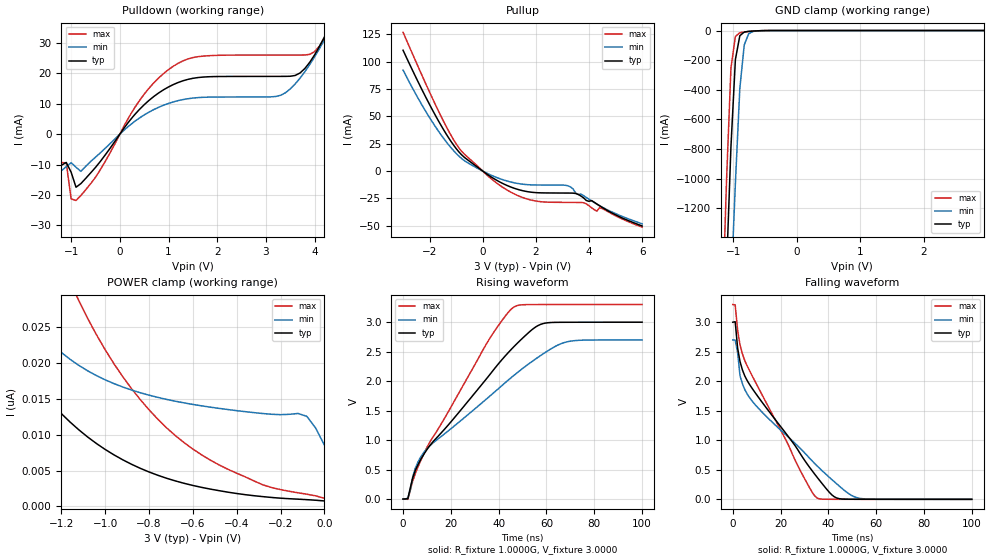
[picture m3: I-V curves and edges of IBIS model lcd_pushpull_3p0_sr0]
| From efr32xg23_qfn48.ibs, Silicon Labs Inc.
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|   Model lcd_pushpull_3p0_sr0
[Model]  lcd_pushpull_3p0_sr0
Model_type 3-state
Polarity   Non-Inverting
Enable   Active-High
C_comp   1.6300pF   1.4000pF   2.7000pF
[Temperature Range]   25.0000   0.1250k   -40.0000
[Pullup Reference]   3.0000V   2.7000V   3.3000V
[Pulldown Reference]   0.0V   0.0V   0.0V
[POWER Clamp Reference]   3.0000V   2.7000V   3.3000V
[GND Clamp Reference]   0.0V   0.0V   0.0V
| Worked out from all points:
|   slope of the pulldown table from 0 to 0.45 V, typ, clamps not added: 50.8 ohm
|   slope of the pullup table from 0 to 0.45 V, typ, clamps not added: 61.2 ohm
|   GND clamp passes 1 mA (typ) near -0.56 V on its own axis
|   rising waveform, R_fixture 1.0000G, V_fixture 3.0000: 20-80 % time 35.7ns typ, 43ns min, 27.5ns max; typ from 0 V to 3 V
|   falling waveform, R_fixture 1.0000G, V_fixture 3.0000: 20-80 % time 28.4ns typ, 33.1ns min, 23.2ns max; typ from 3 V to 0 V
[Pulldown]
|Voltage   I(typ)   I(min)   I(max)
-3V       -29.4mA    -32.34mA   -24.51mA
-1.2V     -10.22mA   -12.02mA   -9.329mA
-1.1V     -9.298mA   -10.66mA   -9.429mA
-1V       -12.5mA    -9.381mA   -21.28mA
-900mV    -17.44mA   -10.87mA   -21.78mA
-800mV    -16.24mA   -12.22mA   -20.16mA
500mV     9.663mA    6.314mA    13.13mA
1.3V      17.55mA    11.37mA    24.1mA
3.3V      18.98mA    12.75mA    25.98mA
3.9V      23.59mA    22.85mA    26.21mA
4.4V      38.7mA     37.11mA    38.07mA
6V        113.8mA    103.8mA    120mA
[Pullup]
|Voltage   I(typ)   I(min)   I(max)
-3V       110.5mA    92.37mA    126.9mA
-2V       60.77mA    48.83mA    72.09mA
-1.1V     23.81mA    18.74mA    28.76mA
-700mV    12.76mA    9.696mA    15.64mA
400mV     -6.625mA   -4.651mA   -8.607mA
1.7V      -18.89mA   -12.46mA   -25.74mA
3.2V      -20.11mA   -13.42mA   -28.65mA
3.5V      -20.5mA    -20.09mA   -28.69mA
3.8V      -24.56mA   -22.6mA    -28.98mA
4.3V      -30.18mA   -30.25mA   -36.64mA
4.5V      -33.28mA   -32.98mA   -34.28mA
6V        -50.2mA    -48.25mA   -51.3mA
[GND_clamp]
|Voltage   I(typ)   I(min)   I(max)
-3V       -24.27A    -21.95A    -26.57A
-1.18V    -2.447A    -3.183A    -1.952A
-1.11V    -1.614A    -2.464A    -1.015A
-1.04V    -784mA     -1.746A    -252.8mA
-970mV    -196.2mA   -1.031A    -40.03mA
-900mV    -35mA      -390.7mA   -14.95mA
-830mV    -10.34mA   -96.94mA   -9.948mA
-760mV    -5.711mA   -21.43mA   -6.561mA
-690mV    -3.47mA    -6.05mA    -3.879mA
-340mV    -10.36uA   -45.49uA   -3.3uA
2.95V     657.9pA    12.89nA    538.5pA
[POWER_clamp]
|Voltage   I(typ)   I(min)   I(max)
-3V       338.2nA    9.289uA    586.7nA
-1.56V    29.18nA    39.44nA    70.52nA
-1.4V     20.57nA    28.74nA    51.74nA
-1.28V    15.63nA    23.83nA    40.5nA
-1.12V    10.68nA    19.68nA    28.7nA
-1V       7.945nA    17.67nA    21.86nA
-880mV    5.879nA    16.25nA    16.45nA
-640mV    3.219nA    14.45nA    8.897nA
-280mV    1.357nA    12.96nA    2.997nA
-120mV    1.003nA    12.97nA    1.894nA
-80mV     936.4pA    12.58nA    1.698nA
0V        757.3pA    8.576nA    1.134nA
[Ramp]
| variable   typ   min   max
dV/dt_r  1.7810/38.6720n   1.5858/48.4026n   1.9678/29.1326n
dV/dt_f  1.7893/31.8128n   1.6007/39.1915n   1.9729/24.9987n
R_load = 10.0000k
[Rising Waveform]
R_fixture= 1.0000G
V_fixture= 3.0000
V_fixture_min= 2.7000
V_fixture_max= 3.3000
|time   V(typ)   V(min)   V(max)
0s        214.6uV    425.1uV    123.1uV
2.02ns    8.808mV    17.95mV    -4.717mV
5.051ns   477.2mV    514mV      424.4mV
10.1ns    845.4mV    859.4mV    883.8mV
35.35ns   2.063V     1.713V     2.663V
45.45ns   2.546V     2.067V     3.228V
48.48ns   2.67V      2.166V     3.288V
56.57ns   2.945V     2.407V     3.299V
67.68ns   2.998V     2.657V     3.299V
100ns     2.999V     2.699V     3.3V
[Falling Waveform]
R_fixture= 1.0000G
V_fixture= 3.0000
V_fixture_min= 2.7000
V_fixture_max= 3.3000
|time   V(typ)   V(min)   V(max)
0s        2.999V     2.699V     3.3V
1.01ns    3.008V     2.696V     3.294V
2.02ns    2.566V     2.488V     2.866V
3.03ns    2.334V     2.094V     2.615V
7.071ns   1.942V     1.72V      2.175V
29.29ns   706.9mV    819.6mV    406.9mV
35.35ns   370.5mV    563.7mV    20.96mV
42.42ns   44.63mV    299.9mV    965.8uV
52.53ns   1.317mV    22.28mV    437.8uV
100ns     217.2uV    447uV      123.6uV
